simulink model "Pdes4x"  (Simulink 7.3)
settings: Solver=ode45  StartTime=0.0  StopTime=50  RelTol=1e-3
undefined symbols (not defined in the file or in its folder): Aps, Bps, Cps, Dps, Kmix

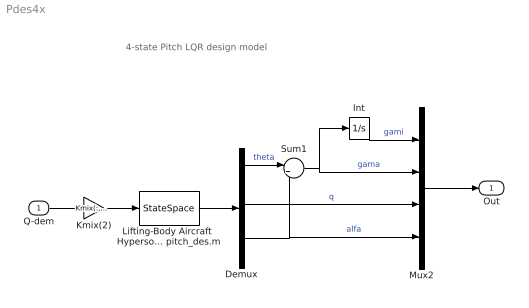
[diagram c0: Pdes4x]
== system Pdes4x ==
  note: 4-state Pitch LQR design model
  Q-dem : Inport  OutDataType=sfix(16)  OutScaling=2^0
  Demux : Demux  Outputs=3
  Int : Integrator
  Kmix(2) : Gain  Gain=Kmix(:,2)  ParameterDataType=sfix(16)  ParameterScaling=2^0  OutDataType=sfix(16)  OutScaling=2^0
  Lifting-Body Aircraft  Hypersonic Pitch  Design Model from file pitch_des.m : StateSpace  A=Aps  B=Bps  C=Cps  D=Dps
  Mux2 : Mux
  Sum1 : Sum  Inputs=|+-  OutDataType=sfix(16)  OutScaling=2^0
  Out : Outport  OutDataType=sfix(16)  OutScaling=2^0
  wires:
  Lifting-Body Aircraft  Hypersonic Pitch  Design Model from file pitch_des.m/1 -> Demux/1
  Demux/2 -> Mux2/3  "q"
  Q-dem/1 -> Kmix(2)/1
  Demux/3 -> Sum1/2, Mux2/4  "alfa"
  Demux/1 -> Sum1/1  "theta"
  Sum1/1 -> Mux2/2, Int/1  "gama"
  Kmix(2)/1 -> Lifting-Body Aircraft  Hypersonic Pitch  Design Model from file pitch_des.m/1
  Int/1 -> Mux2/1  "gami"
  Mux2/1 -> Out/1
